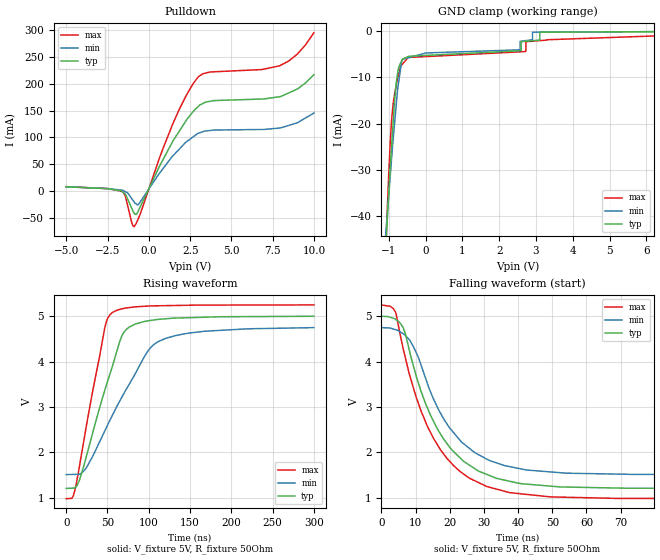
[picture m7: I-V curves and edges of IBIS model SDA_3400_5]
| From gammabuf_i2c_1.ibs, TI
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|   Input/Output open drain SDA_3400 model 5V with 3.4 MHz CLOCK
[Model]   SDA_3400_5
Model_type   I/O_open_drain
|Signals   SDA
| variable   typ   min   max
|C_comp Average
C_comp   8.7291938e-11   7.1019179e-11   1.1120047e-10
|C_comp Output Low
|C_comp   1.7279960e-10   1.4013090e-10   2.2078420e-10
|C_comp Output High
|C_comp   1.7842760e-12   1.9074570e-12   1.6167470e-12
Vinl = 1.5
Vinh = 3.5
Vmeas = 2.5
Vref = 2.5
Cref = 15pF
Rref = 50
[Voltage Range]   5   4.75   5.25
[Temperature Range]   27   85   -40
[Pullup Reference]   5   4.75   5.25
[Pulldown Reference]   0   0   0
[Power Clamp Reference]   5   4.75   5.25
[GND Clamp Reference]   -0   0   0
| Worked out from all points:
|   slope of the pulldown table from 0 to 0.75 V, typ, clamps not added: 15.7 ohm
|   falling waveform, V_fixture 5V, R_fixture 50Ohm: 20-80 % time 13.6ns typ, 13.8ns min, 13.5ns max; typ from 5 V to 1.21 V
|   rising waveform, V_fixture 5V, R_fixture 50Ohm: 20-80 % time 36.3ns typ, 56ns min, 25.9ns max; typ from 1.21 V to 5 V
[Pulldown]
|   Voltage   I(typ)   I(min)   I(max)
-5V       8.33mA     8.229mA    8.568mA
-1.637V   7.48uA     2.021mA    -146.3uA
-1.426V   -5.442mA   -676.3uA   -8.669mA
-1.044V   -30.97mA   -13.28mA   -57.16mA
-897.2mV  -40.15mA   -19.65mA   -65.67mA
-618.4mV  -35.24mA   -24.34mA   -49.57mA
1.429V    91.77mA    64.97mA    123.8mA
2.962V    156.8mA    107.4mA    211.6mA
3.936V    168.5mA    113.7mA    221.9mA
7.892V    175.7mA    117.4mA    232.9mA
8.97V     189.7mA    127mA      254.5mA
9.985V    216.4mA    145.4mA    294.4mA
[GND Clamp]
|   Voltage   I(typ)   I(min)   I(max)
-5V       -668.6mA   -488.5mA   -1.015A
-1.057V   -43.47mA   -41.55mA   -42.51mA
-952.4mV  -28.72mA   -30.73mA   -23.22mA
-869.6mV  -18.59mA   -22.52mA   -15.2mA
-751.9mV  -8.782mA   -12.31mA   -10.05mA
-653.5mV  -6.501mA   -6.808mA   -7.4mA
-449.2mV  -5.455mA   -5.735mA   -5.713mA
2.564V    -4.266mA   -4.058mA   -4.498mA
2.603V    -2.296mA   -2.194mA   -4.482mA
2.913V    -2.08mA    -251.5uA   -2.191mA
3.11V     -257.7uA   -244.5uA   -2.077mA
9.985V    0A         0A         0A
[POWER Clamp]
|   Voltage   I(typ)   I(min)   I(max)
-5V       0A         0A         0A
0V        0A         0A         0A
10V       0A         0A         0A
[Ramp]
R_load = 50
|   typ   min   max
dV/dt_r   2.27599/3.61855e-008   1.94313/5.58979e-008   2.56172/2.58526e-008
dV/dt_f   2.27599/1.35323e-008   1.94313/1.36776e-008   2.56172/1.35215e-008
[Falling Waveform]
V_fixture = 5V
V_fixture_min = 4.75V
V_fixture_max = 5.25V
R_fixture = 50Ohm
C_fixture = 0F
|   Time   V(typ)   V(min)   V(max)
0s        5V         4.75V      5.25V
4.139ns   4.933V     4.706V     5.097V
6.316ns   4.76V      4.62V      4.311V
9.428ns   3.893V     4.324V     3.411V
11.76ns   3.319V     3.895V     2.886V
17.3ns    2.406V     2.866V     2.06V
27.29ns   1.644V     1.997V     1.377V
37.3ns    1.368V     1.691V     1.119V
73.94ns   1.211V     1.516V     985.5mV
300ns     1.207V     1.511V     980.5mV
[Rising Waveform]
V_fixture = 5V
V_fixture_min = 4.75V
V_fixture_max = 5.25V
R_fixture = 50Ohm
C_fixture = 0F
|   Time   V(typ)   V(min)   V(max)
0s        1.207V     1.511V     980.5mV
10.25ns   1.215V     1.516V     1.149V
23.95ns   1.879V     1.651V     2.534V
46.54ns   3.357V     2.466V     4.73V
55.45ns   3.869V     2.798V     5.076V
72.31ns   4.701V     3.377V     5.182V
98.38ns   4.897V     4.218V     5.224V
111.8ns   4.931V     4.444V     5.231V
168.2ns   4.979V     4.671V     5.246V
300ns     5V         4.75V      5.25V
